|   stm32f745_746_756_wlcsp143 IBIS Model
[IBIS ver]   4.2
[File name]  stm32f745_746_756_wlcsp143.ibs
[File Rev]   1.0
[Date]   24-06-2015
[Source] Data Created at STMicroelectronics
[Notes]   File originated from ELDO simulations.
[Disclaimer]  This information is for modeling purpose only and is
   not guaranted. The information is subject to change without
   notice.
[Copyright] Copyright 2015 STMicroelectronics Inc.
[Component] stm32f745_746_756_wlcsp143
[Manufacturer] STMicroelectronics
[Package]
| variable   typ   min   max
R_pkg   0.0   NA   NA
L_pkg   0.0H   NA   NA
C_pkg   0.0F   NA   NA
[Pin]   signal_name   model_name   R_pin   L_pin   C_pin
A1  VDD POWER
A10 PE1 io8p_arsudq_ft
A11 PDR_ON NC
A2 PC10 io8p_arsudq_ft
A3 PD2 io8p_arsudq_ft
A4 PD5 io8p_arsudq_ft
A5 PD7 io8p_arsudq_ft
A6 PG12 io8p_arsudq_ft
A7 PG15 io8p_arsudq_ft
A8 PB6 io8p_arsudq_i2cin_ft
A9 PB8 io8p_arsudq_i2cin_ft
B1 PA14 io8p_arsudq_ft
B10 PE0 io8p_arsudq_ft
B11 PE4 io8p_arsudq_ft
B2 PC11 io8p_arsudq_ft
B3 PD0 io8p_arsudq_ft
B4 PD3 io8p_arsudq_ft
B5 PD4 io8p_arsudq_ft
B6 PG11 io8p_arsudq_ft
B7 PB3 io8p_arsudq_ft
B8 PB7 io8p_arsudq_i2cin_ft
B9 PB9 io8p_arsudq_i2cin_ft
C1 VDD POWER
C10 PE3 io8p_arsudq_ft
C11 VBAT POWER
C2 PA15 io8p_arsudq_ft
C3 PC12 io8p_arsudq_ft
C4 PD1 io8p_arsudq_ft
C5 VDD POWER
C6 PG10 io8p_arsudq_ft
C7 PB4 io8p_arsudq_ft
C8 PB5 io8p_ar3wsudq_ft
C9 BOOT vpp_test_hv
D1  VCAP2 POWER
D10 PC13-ANTI_TAMP io8p_arwsudq_ft_v33
D11 PC14-OSC32_IN io8p_arwsudq_ft_v33
D2 VSS  GND
D3 PA13 io8p_arsudq_ft
D4 PA11 io8usb_lsfs_otg_ft
D5 PA10 io8usb_id_otg_ft
D6 PG13 io8p_arsudq_ft
D7 VDD POWER
D8 PE2 io8p_arsudq_ft
D9 PE5 io8p_arsudq_ft
E1 PA12 io8usb_lsfs_otg_ft
E10 VDD POWER
E11 PC15-OSC32_OUT io8p_arsudq_ft
E2 PA9 io8usb_vbus_otg_ft
E3 PC9 io8p_arsudq_i2cin_ft
E4 PC8 io8p_arsudq_ft
E5 PG9 io8p_arsudq_ft
E6 VDD POWER
E7 VSS GND
E8 PE6 io8p_arsudq_ft
E9 PF1 io8p_arsudq_i2cin_ft
F1 PA8 io8p_arsudq_i2cin_ft
F10 PF2 io8p_arsudq_ft
F11 PF0 io8p_arsudq_i2cin_ft
F2 PC6 io8p_arsudq_ft
F3 PC7 io8p_arsudq_ft
F4 PD6 io8p_arsudq_ft
F5 VSS GND
F6 PG14 io8p_arsudq_ft
F7 PF7 io8p_arwsudq_ft
F8 PF5 io8p_arwsudq_ft
F9 PF4 io8p_arwsudq_ft
G1 VDDUSB POWER
G10 PF6 io8p_arwsudq_ft
G11 PF3 io8p_arwsudq_ft
G2 PG8 io8p_arsudq_ft
G3 PG3 io8p_arsudq_ft
G4 PG6 io8p_arsudq_ft
G5 PG4 io8p_arsudq_ft
G6 PG5 io8p_arsudq_ft
G7 VDD POWER
G8 PF9 io8p_arwsudq_ft
G9 PF10 io8p_arwsudq_ft
H1 PG7 io8p_arsudq_ft
H10 PH1-OSC_OUT io8p_arsudq_ft
H11 PF8 io8p_arwsudq_ft
H2 VSS GND
H3 VSS GND
H4 PD10 io8p_arsudq_ft
H5 PD13 io8p_arsudq_i2cin_ft
H6 PD12 io8p_arsudq_i2cin_ft
H7 VSS GND
H8 PC0 io8p_ar3wsudq_ft
H9 NRST ioreset_ft_v33
J1 PG2 io8p_arsudq_ft
J10 PC2 io8p_ar3wsudq_ft
J11 PH0-OSC_IN io8p_arsudq_ft
J2 PD14 io8p_arsudq_ft
J3 PB15 io8usb_lsfs_otg_ft
J4 PE10 io8p_arsudq_ft
J5 VDD POWER
J6 VDD POWER
J7 VDD POWER
J8 VDD POWER
J9 PC3 io8p_ar3wsudq_ft
K1  PD15 io8p_arsudq_ft
K10 VSSA GND
K11 PC1 io8p_ar3wsudq_ft_v33
K2 PD11 io8p_arsudq_ft
K3 PB14 io8usb_lsfs_otg_ft
K4 PE11 io8p_arsudq_ft
K5 PG1 io8p_arsudq_ft
K6 PF13 io8p_arsudq_ft
K7 PB1 io8p_ar3wsudq_ft
K8 PA1 io8p_ar3wsudq_ft
K9 PA0-WKUP io8p_ar3wsudq_ft_v33
L1 VDD POWER
L10 VDDA POWER
L11 VREF+ POWER
L2 PD8 io8p_arsudq_ft
L3 PE15 io8p_ar3wsudq_ft
L4 PE12 io8p_arsudq_ft
L5 PE7 io8p_arsudq_ft
L6 PF14 io8p_arsudq_i2cin_ft
L7 PB2 io8p_ar3wsudq_ft
L8 PA7 io8p_ar3wsudq_ft
L9 PA2 io8p_ar3wsudq_ft_v33
M1 PD9 io8p_arsudq_ft
M10 PA4 io8p_ar3wsudq_ft
M11 PA3 io8p_ar3wsudq_ft
M2 PB12 io8usb_id_otg_ft
M3 PB10 io8p_arsudq_i2cin_ft
M4 PE14 io8p_arsudq_ft
M5 PE8 io8p_arsudq_ft
M6 PF15 io8p_arsudq_i2cin_ft
M7 PF11 io8p_arsudq_ft
M8 PC4 io8p_ar3wsudq_ft
M9 PA5 io8p_ar3wsudq_ft
N1 PB13 io8usb_vbus_otg_ft
N10 PA6 io8p_ar3wsudq_ft
N11 BYPASS_REG NC
N2 VCAP1 POWER
N3 PB11 io8p_arsudq_i2cin_ft
N4 PE13 io8p_arsudq_ft
N5 PE9 io8p_arsudq_ft
N6 PG0 io8p_arsudq_ft
N7 PF12 io8p_arsudq_ft
N8 PB0 io8p_ar3wsudq_ft
N9 PC5 io8p_ar3wsudq_ft
[Diff Pin]   inv_pin   vdiff   tdelay_typ  tdelay_min  tdelay_max
D4   E1   200mV   NA   NA   NA
J3   K3   200mV   NA   NA   NA
[Model Selector] io8p_ar3wsudq_ft
io8p00_ar3wsudq_ft_pd_lv  "SPEED00 1P8V, PD=40kOhm"
io8p00_ar3wsudq_ft_pu_lv  "SPEED00 1P8V, PU=40kOhm"
io8p00_ar3wsudq_ft_lv  "SPEED00 1P8V"
io8p01_ar3wsudq_ft_pd_lv  "SPEED01 1P8V, PD=40kOhm"
io8p01_ar3wsudq_ft_pu_lv  "SPEED01 1P8V, PU=40kOhm"
io8p01_ar3wsudq_ft_lv  "SPEED01 1P8V"
io8p10_ar3wsudq_ft_pd_lv  "SPEED10 1P8V, PD=40kOhm"
io8p10_ar3wsudq_ft_pu_lv  "SPEED10 1P8V, PU=40kOhm"
io8p10_ar3wsudq_ft_lv  "SPEED10 1P8V"
io8p11_ar3wsudq_ft_pd_lv  "SPEED11 1P8V, PD=40kOhm"
io8p11_ar3wsudq_ft_pu_lv  "SPEED11 1P8V, PU=40kOhm"
io8p11_ar3wsudq_ft_lv  "SPEED11 1P8V"
io8p00_ar3wsudq_ft_pd  "SPEED00, PD=40kOhm"
io8p00_ar3wsudq_ft_pu  "SPEED00, PU=40kOhm"
io8p00_ar3wsudq_ft  "SPEED00"
io8p01_ar3wsudq_ft_pd  "SPEED01, PD=40kOhm"
io8p01_ar3wsudq_ft_pu  "SPEED01, PU=40kOhm"
io8p01_ar3wsudq_ft  "SPEED01"
io8p10_ar3wsudq_ft_pd  "SPEED10, PD=40kOhm"
io8p10_ar3wsudq_ft_pu  "SPEED10, PU=40kOhm"
io8p10_ar3wsudq_ft  "SPEED10"
io8p11_ar3wsudq_ft_pd  "SPEED11, PD=40kOhm"
io8p11_ar3wsudq_ft_pu  "SPEED11, PU=40kOhm"
io8p11_ar3wsudq_ft  "SPEED11"
[Model Selector] io8p_ar3wsudq_ft_v33
io8p00_ar3wsudq_ft_v33_pd_lv  "SPEED00 1P8V, PD=40kOhm"
io8p00_ar3wsudq_ft_v33_pu_lv  "SPEED00 1P8V, PU=40kOhm"
io8p00_ar3wsudq_ft_v33_lv  "SPEED00 1P8V"
io8p01_ar3wsudq_ft_v33_pd_lv  "SPEED01 1P8V, PD=40kOhm"
io8p01_ar3wsudq_ft_v33_pu_lv  "SPEED01 1P8V, PU=40kOhm"
io8p01_ar3wsudq_ft_v33_lv  "SPEED01 1P8V"
io8p10_ar3wsudq_ft_v33_pd_lv  "SPEED10 1P8V, PD=40kOhm"
io8p10_ar3wsudq_ft_v33_pu_lv  "SPEED10 1P8V, PU=40kOhm"
io8p10_ar3wsudq_ft_v33_lv  "SPEED10 1P8V"
io8p11_ar3wsudq_ft_v33_pd_lv  "SPEED11 1P8V, PD=40kOhm"
io8p11_ar3wsudq_ft_v33_pu_lv  "SPEED11 1P8V, PU=40kOhm"
io8p11_ar3wsudq_ft_v33_lv  "SPEED11 1P8V"
io8p00_ar3wsudq_ft_v33_pd  "SPEED00, PD=40kOhm"
io8p00_ar3wsudq_ft_v33_pu  "SPEED00, PU=40kOhm"
io8p00_ar3wsudq_ft_v33  "SPEED00"
io8p01_ar3wsudq_ft_v33_pd  "SPEED01, PD=40kOhm"
io8p01_ar3wsudq_ft_v33_pu  "SPEED01, PU=40kOhm"
io8p01_ar3wsudq_ft_v33  "SPEED01"
io8p10_ar3wsudq_ft_v33_pd  "SPEED10, PD=40kOhm"
io8p10_ar3wsudq_ft_v33_pu  "SPEED10, PU=40kOhm"
io8p10_ar3wsudq_ft_v33  "SPEED10"
io8p11_ar3wsudq_ft_v33_pd  "SPEED11, PD=40kOhm"
io8p11_ar3wsudq_ft_v33_pu  "SPEED11, PU=40kOhm"
io8p11_ar3wsudq_ft_v33  "SPEED11"
[Model Selector] io8p_arsudq_ft
io8p00_arsudq_ft_pd_lv  "SPEED00 1P8V, PD=40kOhm"
io8p00_arsudq_ft_pu_lv  "SPEED00 1P8V, PU=40kOhm"
io8p00_arsudq_ft_lv  "SPEED00 1P8V"
io8p01_arsudq_ft_pd_lv  "SPEED01 1P8V, PD=40kOhm"
io8p01_arsudq_ft_pu_lv  "SPEED01 1P8V, PU=40kOhm"
io8p01_arsudq_ft_lv  "SPEED01 1P8V"
io8p10_arsudq_ft_pd_lv  "SPEED10 1P8V, PD=40kOhm"
io8p10_arsudq_ft_pu_lv  "SPEED10 1P8V, PU=40kOhm"
io8p10_arsudq_ft_lv  "SPEED10 1P8V"
io8p11_arsudq_ft_pd_lv  "SPEED11 1P8V, PD=40kOhm"
io8p11_arsudq_ft_pu_lv  "SPEED11 1P8V, PU=40kOhm"
io8p11_arsudq_ft_lv  "SPEED11 1P8V"
io8p00_arsudq_ft_pd  "SPEED00, PD=40kOhm"
io8p00_arsudq_ft_pu  "SPEED00, PU=40kOhm"
io8p00_arsudq_ft  "SPEED00"
io8p01_arsudq_ft_pd  "SPEED01, PD=40kOhm"
io8p01_arsudq_ft_pu  "SPEED01, PU=40kOhm"
io8p01_arsudq_ft  "SPEED01"
io8p10_arsudq_ft_pd  "SPEED10, PD=40kOhm"
io8p10_arsudq_ft_pu  "SPEED10, PU=40kOhm"
io8p10_arsudq_ft  "SPEED10"
io8p11_arsudq_ft_pd  "SPEED11, PD=40kOhm"
io8p11_arsudq_ft_pu  "SPEED11, PU=40kOhm"
io8p11_arsudq_ft  "SPEED11"
[Model Selector] io8p_arsudq_i2cin_ft
io8p00_arsudq_i2cin_ft_pd_lv  "SPEED00 1P8V, PD=40kOhm"
io8p00_arsudq_i2cin_ft_pu_lv  "SPEED00 1P8V, PU=40kOhm"
io8p00_arsudq_i2cin_ft_lv  "SPEED00 1P8V"
io8p01_arsudq_i2cin_ft_pd_lv  "SPEED01 1P8V, PD=40kOhm"
io8p01_arsudq_i2cin_ft_pu_lv  "SPEED01 1P8V, PU=40kOhm"
io8p01_arsudq_i2cin_ft_lv  "SPEED01 1P8V"
io8p10_arsudq_i2cin_ft_pd_lv  "SPEED10 1P8V, PD=40kOhm"
io8p10_arsudq_i2cin_ft_pu_lv  "SPEED10 1P8V, PU=40kOhm"
io8p10_arsudq_i2cin_ft_lv  "SPEED10 1P8V"
io8p11_arsudq_i2cin_ft_pd_lv  "SPEED11 1P8V, PD=40kOhm"
io8p11_arsudq_i2cin_ft_pu_lv  "SPEED11 1P8V, PU=40kOhm"
io8p11_arsudq_i2cin_ft_lv  "SPEED11 1P8V"
io8p00_arsudq_i2cin_ft_pd  "SPEED00, PD=40kOhm"
io8p00_arsudq_i2cin_ft_pu  "SPEED00, PU=40kOhm"
io8p00_arsudq_i2cin_ft  "SPEED00"
io8p01_arsudq_i2cin_ft_pd  "SPEED01, PD=40kOhm"
io8p01_arsudq_i2cin_ft_pu  "SPEED01, PU=40kOhm"
io8p01_arsudq_i2cin_ft  "SPEED01"
io8p10_arsudq_i2cin_ft_pd  "SPEED10, PD=40kOhm"
io8p10_arsudq_i2cin_ft_pu  "SPEED10, PU=40kOhm"
io8p10_arsudq_i2cin_ft  "SPEED10"
io8p11_arsudq_i2cin_ft_pd  "SPEED11, PD=40kOhm"
io8p11_arsudq_i2cin_ft_pu  "SPEED11, PU=40kOhm"
io8p11_arsudq_i2cin_ft  "SPEED11"
[Model Selector] io8p_arwsudq_ft_v33
io8p00_arwsudq_ft_v33_pd_lv  "SPEED00 1P8V, PD=40kOhm"
io8p00_arwsudq_ft_v33_pu_lv  "SPEED00 1P8V, PU=40kOhm"
io8p00_arwsudq_ft_v33_lv  "SPEED00 1P8V"
io8p01_arwsudq_ft_v33_pd_lv  "SPEED01 1P8V, PD=40kOhm"
io8p01_arwsudq_ft_v33_pu_lv  "SPEED01 1P8V, PU=40kOhm"
io8p01_arwsudq_ft_v33_lv  "SPEED01 1P8V"
io8p10_arwsudq_ft_v33_pd_lv  "SPEED10 1P8V, PD=40kOhm"
io8p10_arwsudq_ft_v33_pu_lv  "SPEED10 1P8V, PU=40kOhm"
io8p10_arwsudq_ft_v33_lv  "SPEED10 1P8V"
io8p11_arwsudq_ft_v33_pd_lv  "SPEED11 1P8V, PD=40kOhm"
io8p11_arwsudq_ft_v33_pu_lv  "SPEED11 1P8V, PU=40kOhm"
io8p11_arwsudq_ft_v33_lv  "SPEED11 1P8V"
io8p00_arwsudq_ft_v33_pd  "SPEED00, PD=40kOhm"
io8p00_arwsudq_ft_v33_pu  "SPEED00, PU=40kOhm"
io8p00_arwsudq_ft_v33  "SPEED00"
io8p01_arwsudq_ft_v33_pd  "SPEED01, PD=40kOhm"
io8p01_arwsudq_ft_v33_pu  "SPEED01, PU=40kOhm"
io8p01_arwsudq_ft_v33  "SPEED01"
io8p10_arwsudq_ft_v33_pd  "SPEED10, PD=40kOhm"
io8p10_arwsudq_ft_v33_pu  "SPEED10, PU=40kOhm"
io8p10_arwsudq_ft_v33  "SPEED10"
io8p11_arwsudq_ft_v33_pd  "SPEED11, PD=40kOhm"
io8p11_arwsudq_ft_v33_pu  "SPEED11, PU=40kOhm"
io8p11_arwsudq_ft_v33  "SPEED11"
[Model Selector] io8usb_id_otg_ft
io8p00_id_otg_ft_pd_lv  "SPEED00 1P8V, PD=14kOhm"
io8p00_id_otg_ft_pu_lv  "SPEED00 1P8V, PU=14kOhm"
io8p00_id_otg_ft_lv  "SPEED00 1P8V"
io8p01_id_otg_ft_pd_lv  "SPEED01 1P8V, PD=14kOhm"
io8p01_id_otg_ft_pu_lv  "SPEED01 1P8V, PU=14kOhm"
io8p01_id_otg_ft_lv  "SPEED01 1P8V"
io8p10_id_otg_ft_pd_lv  "SPEED10 1P8V, PD=14kOhm"
io8p10_id_otg_ft_pu_lv  "SPEED10 1P8V, PU=14kOhm"
io8p10_id_otg_ft_lv  "SPEED10 1P8V"
io8p11_id_otg_ft_pd_lv  "SPEED11 1P8V, PD=14kOhm"
io8p11_id_otg_ft_pu_lv  "SPEED11 1P8V, PU=14kOhm"
io8p11_id_otg_ft_lv  "SPEED11 1P8V"
io8p00_id_otg_ft_pd  "SPEED00, PD=14kOhm"
io8p00_id_otg_ft_pu  "SPEED00, PU=14kOhm"
io8p00_id_otg_ft  "SPEED00"
io8p01_id_otg_ft_pd  "SPEED01, PD=14kOhm"
io8p01_id_otg_ft_pu  "SPEED01, PU=14kOhm"
io8p01_id_otg_ft  "SPEED01"
io8p10_id_otg_ft_pd  "SPEED10, PD=14kOhm"
io8p10_id_otg_ft_pu  "SPEED10, PU=14kOhm"
io8p10_id_otg_ft  "SPEED10"
io8p11_id_otg_ft_pd  "SPEED11, PD=14kOhm"
io8p11_id_otg_ft_pu  "SPEED11, PU=14kOhm"
io8p11_id_otg_ft  "SPEED11"
[Model Selector] io8usb_lsfs_otg_ft
io8usb_ls_otg_ft_dpdn_pd  "LS USB DP/DN IO + PD=20kOhm"
io8usb_ls_otg_ft_dpdn_pupu2  "LS USB DP/DN IO + PU/PU2=2.2kOhm"
io8usb_ls_otg_ft_dpdn_pu2  "LS USB DP/DN IO + PU2=1.2kOhm"
io8usb_ls_otg_ft_dpdn_pu  "LS USB DP/DN IO + PU=1.2kOhm"
io8usb_ls_otg_ft_dpdn  "LS USB DP/DN IO"
io8usb_fs_otg_ft_dpdn_pd  "HS USB DP/DN IO + PD=20kOhm"
io8usb_fs_otg_ft_dpdn_pupu2  "HS USB DP/DN IO + PU/PU2=2.2kOhm"
io8usb_fs_otg_ft_dpdn_pu2  "HS USB DP/DN IO + PU2=1.2kOhm"
io8usb_fs_otg_ft_dpdn_pu  "HS USB DP/DN IO + PU=1.2kOhm"
io8usb_fs_otg_ft_dpdn  "HS USB DP/DN IO"
io8p00_lsfs_otg_ft_pd_lv  "SPEED00 1P8V, PD=40kOhm"
io8p00_lsfs_otg_ft_pu_lv  "SPEED00 1P8V, PU=40kOhm"
io8p00_lsfs_otg_ft_lv  "SPEED00 1P8V"
io8p01_lsfs_otg_ft_pd_lv  "SPEED01 1P8V, PD=40kOhm"
io8p01_lsfs_otg_ft_pu_lv  "SPEED01 1P8V, PU=40kOhm"
io8p01_lsfs_otg_ft_lv  "SPEED01 1P8V"
io8p10_lsfs_otg_ft_pd_lv  "SPEED10 1P8V, PD=40kOhm"
io8p10_lsfs_otg_ft_pu_lv  "SPEED10 1P8V, PU=40kOhm"
io8p10_lsfs_otg_ft_lv  "SPEED10 1P8V"
io8p11_lsfs_otg_ft_pd_lv  "SPEED11 1P8V, PD=40kOhm"
io8p11_lsfs_otg_ft_pu_lv  "SPEED11 1P8V, PU=40kOhm"
io8p11_lsfs_otg_ft_lv  "SPEED11 1P8V"
io8p00_lsfs_otg_ft_pd  "SPEED00, PD=40kOhm"
io8p00_lsfs_otg_ft_pu  "SPEED00, PU=40kOhm"
io8p00_lsfs_otg_ft  "SPEED00"
io8p01_lsfs_otg_ft_pd  "SPEED01, PD=40kOhm"
io8p01_lsfs_otg_ft_pu  "SPEED01, PU=40kOhm"
io8p01_lsfs_otg_ft  "SPEED01"
io8p10_lsfs_otg_ft_pd  "SPEED10, PD=40kOhm"
io8p10_lsfs_otg_ft_pu  "SPEED10, PU=40kOhm"
io8p10_lsfs_otg_ft  "SPEED10"
io8p11_lsfs_otg_ft_pd  "SPEED11, PD=40kOhm"
io8p11_lsfs_otg_ft_pu  "SPEED11, PU=40kOhm"
io8p11_lsfs_otg_ft  "SPEED11"
[Model Selector] io8usb_vbus_otg_ft
io8psenb_vbus_otg_ft  "VBUS PULSE, SENSE VB"
io8psenab_vbus_otg_ft  "VBUS PULSE, SENSE VA and VB"
io8psena_vbus_otg_ft  "VBUS PULSE, SENSE VA"
io8psen_vbus_otg_ft  "VBUS PULSE"
io8p00_vbus_otg_ft_pd_lv  "SPEED00 1P8V, PD=40kOhm"
io8p00_vbus_otg_ft_pu_lv  "SPEED00 1P8V, PU=40kOhm"
io8p00_vbus_otg_ft_lv  "SPEED00 1P8V"
io8p01_vbus_otg_ft_pd_lv  "SPEED01 1P8V, PD=40kOhm"
io8p01_vbus_otg_ft_pu_lv  "SPEED01 1P8V, PU=40kOhm"
io8p01_vbus_otg_ft_lv  "SPEED01 1P8V"
io8p10_vbus_otg_ft_pd_lv  "SPEED10 1P8V, PD=40kOhm"
io8p10_vbus_otg_ft_pu_lv  "SPEED10 1P8V, PU=40kOhm"
io8p10_vbus_otg_ft_lv  "SPEED10 1P8V"
io8p11_vbus_otg_ft_pd_lv  "SPEED11 1P8V, PD=40kOhm"
io8p11_vbus_otg_ft_pu_lv  "SPEED11 1P8V, PU=40kOhm"
io8p11_vbus_otg_ft_lv  "SPEED11 1P8V"
io8p00_vbus_otg_ft_pd  "SPEED00, PD=40kOhm"
io8p00_vbus_otg_ft_pu  "SPEED00, PU=40kOhm"
io8p00_vbus_otg_ft  "SPEED00"
io8p01_vbus_otg_ft_pd  "SPEED01, PD=40kOhm"
io8p01_vbus_otg_ft_pu  "SPEED01, PU=40kOhm"
io8p01_vbus_otg_ft  "SPEED01"
io8p10_vbus_otg_ft_pd  "SPEED10, PD=40kOhm"
io8p10_vbus_otg_ft_pu  "SPEED10, PU=40kOhm"
io8p10_vbus_otg_ft  "SPEED10"
io8p11_vbus_otg_ft_pd  "SPEED11, PD=40kOhm"
io8p11_vbus_otg_ft_pu  "SPEED11, PU=40kOhm"
io8p11_vbus_otg_ft  "SPEED11"
[Model Selector] ioreset_ft_v33
ioreset_ft_v33_pu_lv  "ioreset 1P8V + PU=40kOhm"
ioreset_ft_v33_nopu_lv  "ioreset 1P8V"
ioreset_ft_v33_pu  "ioreset + PU=40kOhm"
ioreset_ft_v33_nopu  "ioreset"
[Model Selector] vpp_test_hv
vpp_test_hv_2p4  "Input Buffer 1P8V"
vpp_test_hv_3p3  "Input Buffer"
[Model Selector] io8p_arwsudq_ft
io8p00_arwsudq_ft_pd_lv  "SPEED00 1P8V, PD=40kOhm"
io8p00_arwsudq_ft_pu_lv  "SPEED00 1P8V, PU=40kOhm"
io8p00_arwsudq_ft_lv  "SPEED00 1P8V"
io8p01_arwsudq_ft_pd_lv  "SPEED01 1P8V, PD=40kOhm"
io8p01_arwsudq_ft_pu_lv  "SPEED01 1P8V, PU=40kOhm"
io8p01_arwsudq_ft_lv  "SPEED01 1P8V"
io8p10_arwsudq_ft_pd_lv  "SPEED10 1P8V, PD=40kOhm"
io8p10_arwsudq_ft_pu_lv  "SPEED10 1P8V, PU=40kOhm"
io8p10_arwsudq_ft_lv  "SPEED10 1P8V"
io8p11_arwsudq_ft_pd_lv  "SPEED11 1P8V, PD=40kOhm"
io8p11_arwsudq_ft_pu_lv  "SPEED11 1P8V, PU=40kOhm"
io8p11_arwsudq_ft_lv  "SPEED11 1P8V"
io8p00_arwsudq_ft_pd  "SPEED00, PD=40kOhm"
io8p00_arwsudq_ft_pu  "SPEED00, PU=40kOhm"
io8p00_arwsudq_ft  "SPEED00"
io8p01_arwsudq_ft_pd  "SPEED01, PD=40kOhm"
io8p01_arwsudq_ft_pu  "SPEED01, PU=40kOhm"
io8p01_arwsudq_ft  "SPEED01"
io8p10_arwsudq_ft_pd  "SPEED10, PD=40kOhm"
io8p10_arwsudq_ft_pu  "SPEED10, PU=40kOhm"
io8p10_arwsudq_ft  "SPEED10"
io8p11_arwsudq_ft_pd  "SPEED11, PD=40kOhm"
io8p11_arwsudq_ft_pu  "SPEED11, PU=40kOhm"
io8p11_arwsudq_ft  "SPEED11"
| Models and submodels in the file (236): io8p00_ar3wsudq_ft_pd_lv (I/O), io8p00_ar3wsudq_ft_pu_lv (I/O), io8p00_ar3wsudq_ft_lv (I/O), io8p01_ar3wsudq_ft_pd_lv (I/O), io8p01_ar3wsudq_ft_pu_lv (I/O), io8p01_ar3wsudq_ft_lv (I/O), io8p10_ar3wsudq_ft_pd_lv (I/O), io8p10_ar3wsudq_ft_pu_lv (I/O), io8p10_ar3wsudq_ft_lv (I/O), io8p11_ar3wsudq_ft_pd_lv (I/O), io8p11_ar3wsudq_ft_pu_lv (I/O), io8p11_ar3wsudq_ft_lv (I/O), io8p00_ar3wsudq_ft_pd (I/O), io8p00_ar3wsudq_ft_pu (I/O), io8p00_ar3wsudq_ft (I/O), io8p01_ar3wsudq_ft_pd (I/O), io8p01_ar3wsudq_ft_pu (I/O), io8p01_ar3wsudq_ft (I/O), io8p10_ar3wsudq_ft_pd (I/O), io8p10_ar3wsudq_ft_pu (I/O), io8p10_ar3wsudq_ft (I/O), io8p11_ar3wsudq_ft_pd (I/O), io8p11_ar3wsudq_ft_pu (I/O), io8p11_ar3wsudq_ft (I/O), io8p00_ar3wsudq_ft_v33_pd_lv (I/O), io8p00_ar3wsudq_ft_v33_pu_lv (I/O), io8p00_ar3wsudq_ft_v33_lv (I/O), io8p01_ar3wsudq_ft_v33_pd_lv (I/O), io8p01_ar3wsudq_ft_v33_pu_lv (I/O), io8p01_ar3wsudq_ft_v33_lv (I/O), io8p10_ar3wsudq_ft_v33_pd_lv (I/O), io8p10_ar3wsudq_ft_v33_pu_lv (I/O), io8p10_ar3wsudq_ft_v33_lv (I/O), io8p11_ar3wsudq_ft_v33_pd_lv (I/O), io8p11_ar3wsudq_ft_v33_pu_lv (I/O), io8p11_ar3wsudq_ft_v33_lv (I/O), io8p00_ar3wsudq_ft_v33_pd (I/O), io8p00_ar3wsudq_ft_v33_pu (I/O), io8p00_ar3wsudq_ft_v33 (I/O), io8p01_ar3wsudq_ft_v33_pd (I/O), io8p01_ar3wsudq_ft_v33_pu (I/O), io8p01_ar3wsudq_ft_v33 (I/O), io8p10_ar3wsudq_ft_v33_pd (I/O), io8p10_ar3wsudq_ft_v33_pu (I/O), io8p10_ar3wsudq_ft_v33 (I/O), io8p11_ar3wsudq_ft_v33_pd (I/O), io8p11_ar3wsudq_ft_v33_pu (I/O), io8p11_ar3wsudq_ft_v33 (I/O), io8p00_arsudq_ft_pd_lv (I/O), io8p00_arsudq_ft_pu_lv (I/O), io8p00_arsudq_ft_lv (I/O), io8p01_arsudq_ft_pd_lv (I/O), io8p01_arsudq_ft_pu_lv (I/O), io8p01_arsudq_ft_lv (I/O), io8p10_arsudq_ft_pd_lv (I/O), io8p10_arsudq_ft_pu_lv (I/O), io8p10_arsudq_ft_lv (I/O), io8p11_arsudq_ft_pd_lv (I/O), io8p11_arsudq_ft_pu_lv (I/O), io8p11_arsudq_ft_lv (I/O), io8p00_arsudq_ft_pd (I/O), io8p00_arsudq_ft_pu (I/O), io8p00_arsudq_ft (I/O), io8p01_arsudq_ft_pd (I/O), io8p01_arsudq_ft_pu (I/O), io8p01_arsudq_ft (I/O), io8p10_arsudq_ft_pd (I/O), io8p10_arsudq_ft_pu (I/O), io8p10_arsudq_ft (I/O), io8p11_arsudq_ft_pd (I/O), io8p11_arsudq_ft_pu (I/O), io8p11_arsudq_ft (I/O), io8p00_arsudq_i2cin_ft_pd_lv (I/O), io8p00_arsudq_i2cin_ft_pu_lv (I/O), io8p00_arsudq_i2cin_ft_lv (I/O), io8p01_arsudq_i2cin_ft_pd_lv (I/O), io8p01_arsudq_i2cin_ft_pu_lv (I/O), io8p01_arsudq_i2cin_ft_lv (I/O), io8p10_arsudq_i2cin_ft_pd_lv (I/O), io8p10_arsudq_i2cin_ft_pu_lv (I/O)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
